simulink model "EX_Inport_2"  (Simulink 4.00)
settings: Solver=ode45  StartTime=0.0  StopTime=10  FixedStep=0.4  MaxStep=0.01  RelTol=1e-3

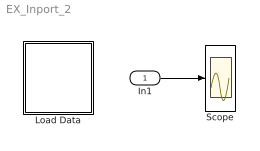
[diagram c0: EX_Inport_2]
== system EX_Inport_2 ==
  In1 : Inport  Port=1  LatchInput=off
  Load Data : Subsystem
  Scope : Scope
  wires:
  In1/1 -> Scope/1

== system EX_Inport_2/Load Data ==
